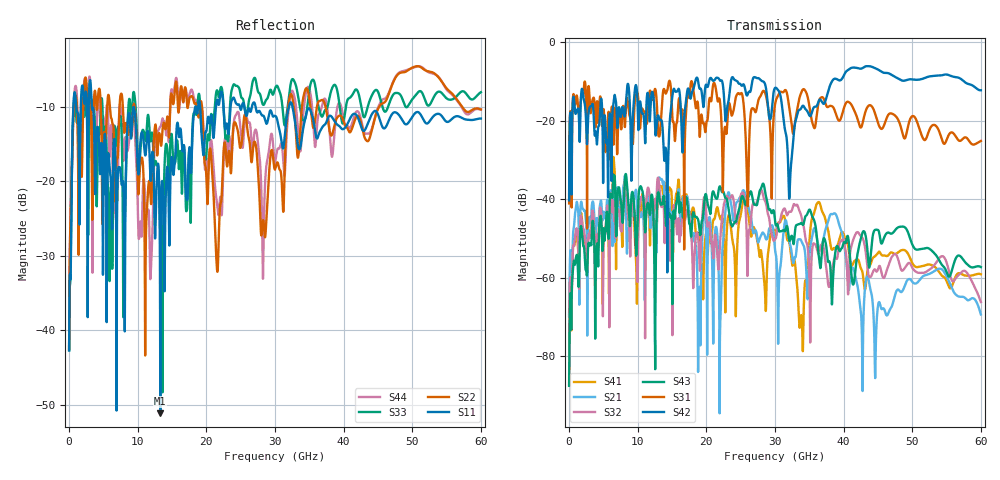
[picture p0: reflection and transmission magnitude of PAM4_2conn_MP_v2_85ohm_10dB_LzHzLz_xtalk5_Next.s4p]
! Info: Touchstone file created by Circ.  Input file=FAB50GbE_2conn_Midplane_Examax_Topo2_v2_85ohm_10dB_LzHzLz.circ
# Hz S RI R 50
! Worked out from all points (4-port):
!   6000 points, 10 MHz to 60 GHz, reference 50 ohm
!   strongest paths, dB at 10 MHz, 15.01 GHz, 30.01 GHz, 45.01 GHz, 60 GHz:
!     S42: -40.3, -14.5, -11.7, -7.0, -12.3
!     S31: -41.1, -18.0, -15.9, -20.6, -25.2
!     S43: -87.5, -52.1, -45.4, -47.8, -57.3
!     S32: -69.8, -53.9, -50.2, -57.8, -66.2
!     S21: -69.3, -46.7, -52.9, -67.1, -69.4
!     S41: -87.2, -42.1, -48.3, -53.7, -59.1
!   lowest |S11| = -51.1 dB at 13.29 GHz (marker M1), VSWR 1.01, Z = 49.9 + j0.255 ohm
!   |S11| at or under -10 dB: 3.319 GHz to 18.38 GHz (15.06 GHz wide, 139 % of centre); 27.18 GHz to 32.03 GHz (4.849 GHz wide, 16.4 % of centre); 32.56 GHz to end of sweep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
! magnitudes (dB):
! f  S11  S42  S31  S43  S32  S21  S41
! 10 MHz  -42.7  -40.3  -41.1  -87.5  -69.8  -69.3  -87.2
! 13.29 GHz  -51.1  -19.9  -22.3  -41.1  -39.2  -34.9  -36.7
! 18.96 GHz  -9.2  -11.6  -21.6  -47.1  -54.6  -62.4  -51.1
! 25.43 GHz  -9.6  -10.8  -15.8  -39.9  -38.7  -37.8  -39.5
! 33.83 GHz  -14.7  -16.8  -12.9  -46.1  -44.3  -50.6  -69.5
! 36.28 GHz  -14.0  -15.5  -16.1  -52.9  -53.8  -51.4  -40.8
! 60 GHz  -11.6  -12.3  -25.2  -57.3  -66.2  -69.4  -59.1
